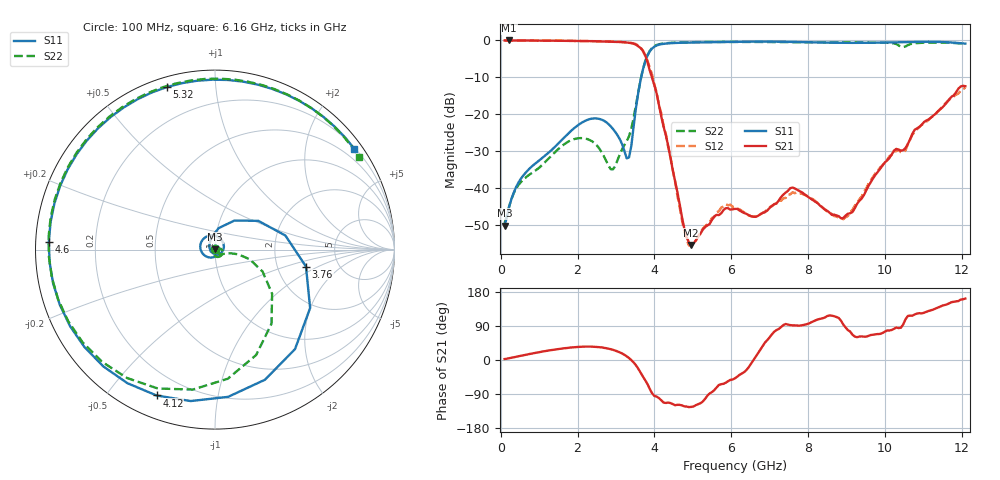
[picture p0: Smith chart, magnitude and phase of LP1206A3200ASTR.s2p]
! File saved on Sunday, September 22, 2019 using DaVinci by Abstraction Software Inc. (c) 1998
# HZ S DB  R 50
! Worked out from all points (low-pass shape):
!   201 points, 100 MHz to 12.1 GHz, reference 50 ohm
!   highest |S21| = -0.01 dB at 220 MHz (marker M1); lowest = -55.4 dB at 4.96 GHz (marker M2)
!   |S21| within 3 dB of the highest: start of sweep to 3.713 GHz
!   lowest |S11| = -50.1 dB at 100 MHz (marker M3), VSWR 1.01, Z = 50.2 + j0.264 ohm
!   |S11| at or under -10 dB: start of sweep to 3.656 GHz
!   |S22| runs from -49.4 to -0.4 dB; largest |S21 - S12| = 0.038
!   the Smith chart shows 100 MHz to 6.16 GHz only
!   S11 on the Smith chart (normalised r, x): 100 MHz: 1.00, +0.01; 3.76 GHz: 2.91, -0.75; 4.12 GHz: 0.10, -0.67; 4.6 GHz: 0.04, +0.02; 5.32 GHz: 0.04, +0.75; 6.16 GHz: 0.22, +3.06
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1e8  -50.11 57.6  -0.01 2.6  -0.01 2.6  -49.42 44.1
2.2e8  -44.94 57.4  -0.01 4.7  -0.01 4.7  -44.85 45.0
6.4e8  -35.91 20.3  -0.04 13.6  -0.03 13.6  -37.19 18.0
2.14e9  -22.09 -176.6  -0.16 35.1  -0.16 35.1  -26.46 -46.2
2.92e9  -23.94 52.3  -0.35 27.0  -0.29 27.1  -34.91 -72.0
3.34e9  -31.67 -152.7  -0.63 5.1  -0.61 5.3  -25.96 -29.6
3.64e9  -10.76 33.5  -2.07 -33.1  -1.86 -33.2  -10.70 -24.8
3.76e9  -5.75 -10.5  -3.97 -53.0  -4.13 -55.9  -5.68 -52.7
3.94e9  -2.20 -69.0  -10.11 -87.8  -9.27 -84.3  -2.05 -99.0
4.12e9  -1.15 -111.8  -17.48 -100.5  -17.45 -107.1  -1.04 -135.2
4.6e9  -0.66 177.2  -41.08 -118.3  -42.02 -119.0  -0.58 162.6
4.96e9  -0.56 139.6  -55.37 -123.8  -55.71 -119.6  -0.48 128.5
5.32e9  -0.50 106.5  -50.56 -102.7  -50.36 -103.1  -0.43 98.2
6.1e9  -0.38 40.9  -45.61 -48.2  -45.04 -52.2  -0.41 37.1
6.16e9  -0.37 36.0  -45.61 -44.0  -45.51 -48.8  -0.41 32.5
6.94e9  -0.32 -24.3  -46.06 52.5  -45.81 47.9  -0.43 -25.6
7.6e9  -0.41 -71.3  -39.83 91.4  -41.12 92.6  -0.47 -72.9
8.14e9  -0.54 -107.8  -43.32 102.4  -43.04 106.4  -0.47 -109.5
9.16e9  -0.66 -174.2  -46.45 66.5  -45.85 66.2  -0.54 -175.5
1.012e10  -0.54 127.3  -31.86 77.9  -31.34 77.2  -0.67 123.1
1.108e10  -0.36 69.3  -21.68 127.1  -22.01 125.0  -0.59 68.1
1.21e10  -0.87 -4.3  -12.40 162.1  -12.77 157.8  -0.92 -3.4
